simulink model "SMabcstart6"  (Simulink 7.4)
settings: Solver=ode45  StartTime=0.0  StopTime=10  MaxStep=2e-4  RelTol=1e-3
InitFcn:
  | smparamstart6
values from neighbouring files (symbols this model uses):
  Bm = 0.10    (= 0.1)    [IMabc2.m]    (also in imabcparam.m = 0.01; IMabcrun0.m = 0.01; IMabcrun1.m = 0.001; IMcur0.m = 1e-06)
  D = str2num(get(h,'string'))    [acttrcalc1.m]
  gam = 2*pi/3    (= 2.09439510239)    [IMabc2.m]    (also in IMabcf0.m; IMabcf1.m; imabcparam.m; IMabcrun0.m)
  H = 0.60    (= 0.6)    [IMabc2.m]    (also in IMcur0.m = 0.3; imdef0vec.m = 0.3; imdef1vec.m = 0.3; imdef2vec.m = 0.3)
  Lrr = [Lr   -Lm/2 -Lm/2    [IMabc2.m]    (also in IMabcf0.m = [Lr   -Lm1/2 -Lm1/2; IMabcf1.m = [Lr   -Lm1/2 -Lm1/2)
  Vm = Vll*sqrt(2/3)    [imabcparam.m]
  wo = 2*pi*freq0    [calc0.m]    (also in IMabc2.m = 376.991118431; imabcparam.m = 376.991118431; IMabcrun0.m = 376.991118431; IMabcrun1.m = 376.991118431)
undefined symbols (not defined in the file or in its folder): L2, Labo, Laf, Lakd, Lakq, Lao, R1, R2, Row, TL1, TL2, vector

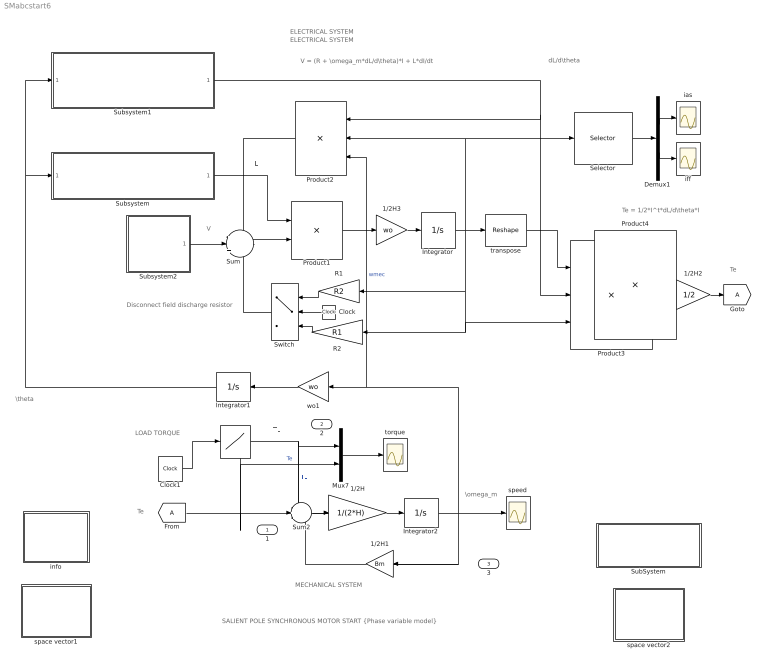
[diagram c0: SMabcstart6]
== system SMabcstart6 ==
  note: I
  note: I'
  note: MECHANICAL SYSTEM
  note: ELECTRICAL SYSTEM
  note: V
  note: SALIENT POLE SYNCHRONOUS MOTOR START {Phase variable model}
  note: L
  note: Te
  note: TL
  note: Te
  note: LOAD TORQUE
  note: Disconnect field discharge resistor
  note: dL/d\theta
  note: ELECTRICAL SYSTEM
  note: V = (R + \omega_m*dL/d\theta)*I + L*dI/dt
  note: \omega_m
  note: \theta
  note: Te = 1/2*I^t*dL/d\theta*I
  " " : Lookup  InputValues=[0 8 8 10 ]  Table="[TL1 TL1  TL2  TL2]"  OutDataType=sfix(16)  OutScaling=2^0
  1/2H : Gain  Gain=1/(2*H)  ParameterDataType=sfix(16)  ParameterScaling=2^0  OutDataType=sfix(16)  OutScaling=2^0
  1/2H1 : Gain  Gain=Bm  ParameterDataType=sfix(16)  ParameterScaling=2^0  OutDataType=sfix(16)  OutScaling=2^0
  1/2H2 : Gain  Gain=1/2  ParameterDataType=sfix(16)  ParameterScaling=2^0  OutDataType=sfix(16)  OutScaling=2^0
  1/2H3 : Gain  Gain=wo  ParameterDataType=sfix(16)  ParameterScaling=2^0  OutDataType=sfix(16)  OutScaling=2^0
  Clock : Clock
  Clock1 : Clock
  Demux1 : Demux  Outputs=2
  Integrator : Integrator  InitialCondition=[0 ;0 ;0; 0 ;0 ;0]
  Integrator1 : Integrator
  Integrator2 : Integrator
  Mux7 : Mux  Inputs=2
  Product1 : Product  Inputs=/*  Multiplication=Matrix(*)  OutDataType=sfix(16)  OutScaling=2^0
  Product2 : Product  Inputs=***  Multiplication=Matrix(*)  OutDataType=sfix(16)  OutScaling=2^0
  Product3 : Product  Inputs=3  Multiplication=Matrix(*)  OutDataType=sfix(16)  OutScaling=2^0
  Product4 : Product  Inputs=3  Multiplication=Matrix(*)  OutDataType=sfix(16)  OutScaling=2^0
  R1 : Gain  Gain=R2  Multiplication=Matrix(K*u)  ParameterDataType=sfix(16)  ParameterScaling=2^0  OutDataType=sfix(16)  OutScaling=2^0
  R2 : Gain  Gain=R1  Multiplication=Matrix(K*u)  ParameterDataType=sfix(16)  ParameterScaling=2^0  OutDataType=sfix(16)  OutScaling=2^0
  Selector : Selector  InputPortWidth=6  IndexOptions=Index vector (dialog)  Indices=[1 4]  OutputSizes=1
  SubSystem : Subsystem
  Subsystem : Subsystem
  Subsystem1 : Subsystem
  Subsystem2 : Subsystem
  Sum : Sum  Inputs=-|+|-  OutDataType=sfix(16)  OutScaling=2^0
  Sum2 : Sum  Inputs=-+-  OutDataType=sfix(16)  OutScaling=2^0
  Switch : Switch  Threshold=4
  ias : Scope
  iff : Scope
  info : Subsystem
  space vector1 : Subsystem
  space vector2 : Subsystem
  speed : Scope
  torque : Scope
  transpose : Reshape  OutputDimensionality=Row vector (2-D)  OutputDimensions=[1,6]
  wo1 : Gain  Gain=wo  ParameterDataType=sfix(16)  ParameterScaling=2^0  OutDataType=sfix(16)  OutScaling=2^0
  1 : Outport
  2 : Outport  Port=2
  3 : Outport  Port=3
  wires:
  Product1/1 -> 1/2H3/1
  Sum/1 -> Product1/2
  transpose/1 -> Product3/1
  Product2/1 -> Sum/1
  Subsystem1/1(dLdtheta) -> Product2/1, Product3/2
  Product3/1 -> 1/2H2/1
  Sum2/1 -> 1/2H/1
  1/2H/1 -> Integrator2/1
  1/2H1/1 -> Sum2/3
  Mux7/1 -> torque/1
  " "/1 -> Mux7/1, Sum2/1, 2/1  "TL"
  [A] -> Sum2/2, 1/1, Mux7/2  "Te"
  Integrator2/1 -> Product2/3, wo1/1, speed/1, 1/2H1/1, 3/1  "wmec"
  Subsystem2/1(V) -> Sum/2
  Integrator1/1 -> Subsystem1/1(theta1), Subsystem/1(theta)
  Clock1/1 -> " "/1
  1/2H2/1 -> [A]
  Subsystem/1(L) -> Product1/1
  R2/1 -> Switch/3
  R1/1 -> Switch/1
  Clock/1 -> Switch/2
  Switch/1 -> Sum/3
  Integrator/1 -> transpose/1, Product2/2, Selector/1, Product3/3, R2/1, R1/1
  Selector/1 -> Demux1/1
  Demux1/2 -> iff/1
  Demux1/1 -> ias/1
  1/2H3/1 -> Integrator/1
  wo1/1 -> Integrator1/1

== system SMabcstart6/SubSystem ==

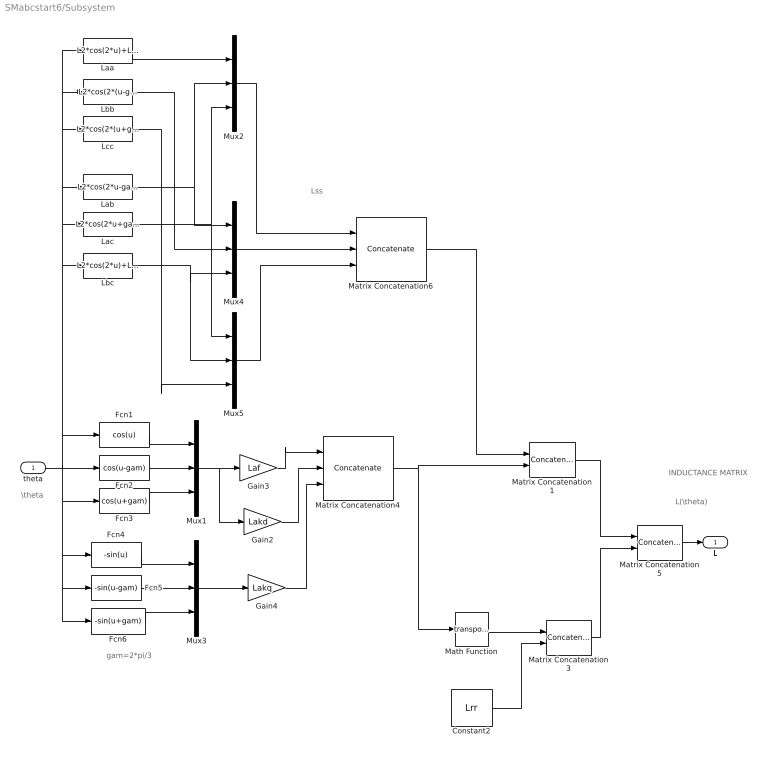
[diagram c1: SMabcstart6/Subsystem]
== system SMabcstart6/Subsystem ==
  note: INDUCTANCE MATRIX
  note: Lss
  note: L(\theta)
  note: gam=2*pi/3
  note: \theta
  theta : Inport  OutDataType=sfix(16)  OutScaling=2^0
  Constant2 : Constant  Value=Lrr  VectorParams1D=off  OutDataType=sfix(16)  OutScaling=2^0
  Fcn1 : Fcn  Expr=cos(u)
  Fcn2 : Fcn  Expr=cos(u-gam)
  Fcn3 : Fcn  Expr=cos(u+gam)
  Fcn4 : Fcn  Expr=-sin(u)
  Fcn5 : Fcn  Expr=-sin(u-gam)
  Fcn6 : Fcn  Expr=-sin(u+gam)
  Gain2 : Gain  Gain=Lakd  ParameterDataType=sfix(16)  ParameterScaling=2^0  OutDataType=sfix(16)  OutScaling=2^0
  Gain3 : Gain  Gain=Laf  ParameterDataType=sfix(16)  ParameterScaling=2^0  OutDataType=sfix(16)  OutScaling=2^0
  Gain4 : Gain  Gain=Lakq  ParameterDataType=sfix(16)  ParameterScaling=2^0  OutDataType=sfix(16)  OutScaling=2^0
  Laa : Fcn  Expr=L2*cos(2*u)+Lao
  Lab : Fcn  Expr=L2*cos(2*u-gam)+Labo
  Lac : Fcn  Expr=L2*cos(2*u+gam)+Labo
  Lbb : Fcn  Expr=L2*cos(2*(u-gam))+Lao
  Lbc : Fcn  Expr=L2*cos(2*u)+Labo
  Lcc : Fcn  Expr=L2*cos(2*(u+gam))+Lao
  Math Function : Math  Operator=transpose
  Matrix Concatenation1 : Concatenate  Mode=Multidimensional array  ConcatenateDimension=2
  Matrix Concatenation3 : Concatenate  Mode=Multidimensional array  ConcatenateDimension=2
  Matrix Concatenation4 : Concatenate  NumInputs=3  Mode=Multidimensional array  ConcatenateDimension=2
  Matrix Concatenation5 : Concatenate  Mode=Multidimensional array
  Matrix Concatenation6 : Concatenate  NumInputs=3  Mode=Multidimensional array  ConcatenateDimension=2
  Mux{1..5} (5 alike) : Mux  Inputs=3
  L : Outport
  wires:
  Matrix Concatenation5/1 -> L/1
  Matrix Concatenation4/1 -> Matrix Concatenation1/2, Math Function/1
  Mux1/1 -> Gain3/1, Gain2/1
  Matrix Concatenation1/1 -> Matrix Concatenation5/1
  Fcn3/1 -> Mux1/3
  Fcn2/1 -> Mux1/2
  Fcn1/1 -> Mux1/1
  theta/1 -> Fcn2/1, Fcn3/1, Fcn6/1, Fcn5/1, Fcn4/1, Fcn1/1, Laa/1, Lbb/1, Lcc/1, Lab/1, Lac/1, Lbc/1
  Gain3/1 -> Matrix Concatenation4/1
  Gain2/1 -> Matrix Concatenation4/2
  Fcn5/1 -> Mux3/2
  Fcn4/1 -> Mux3/1
  Fcn6/1 -> Mux3/3
  Mux3/1 -> Gain4/1
  Gain4/1 -> Matrix Concatenation4/3
  Constant2/1 -> Matrix Concatenation3/2
  Matrix Concatenation3/1 -> Matrix Concatenation5/2
  Laa/1 -> Mux2/1
  Lbb/1 -> Mux4/2
  Lab/1 -> Mux2/2, Mux4/1
  Lac/1 -> Mux2/3, Mux5/1
  Lbc/1 -> Mux4/3, Mux5/2
  Lcc/1 -> Mux5/3
  Mux4/1 -> Matrix Concatenation6/2
  Mux2/1 -> Matrix Concatenation6/1
  Mux5/1 -> Matrix Concatenation6/3
  Matrix Concatenation6/1 -> Matrix Concatenation1/1
  Math Function/1 -> Matrix Concatenation3/1

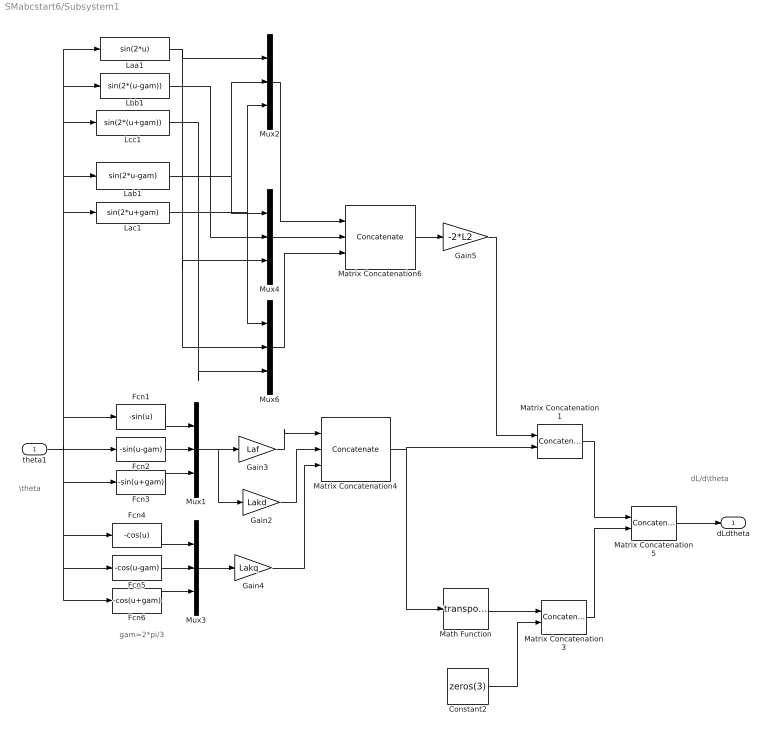
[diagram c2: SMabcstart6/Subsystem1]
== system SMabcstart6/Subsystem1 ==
  note: dL/d\theta
  note: \theta
  note: gam=2*pi/3
  theta1 : Inport  OutDataType=sfix(16)  OutScaling=2^0
  Constant2 : Constant  Value=zeros(3)  VectorParams1D=off  OutDataType=sfix(16)  OutScaling=2^0
  Fcn1 : Fcn  Expr=-sin(u)
  Fcn2 : Fcn  Expr=-sin(u-gam)
  Fcn3 : Fcn  Expr=-sin(u+gam)
  Fcn4 : Fcn  Expr=-cos(u)
  Fcn5 : Fcn  Expr=-cos(u-gam)
  Fcn6 : Fcn  Expr=-cos(u+gam)
  Gain2 : Gain  Gain=Lakd  ParameterDataType=sfix(16)  ParameterScaling=2^0  OutDataType=sfix(16)  OutScaling=2^0
  Gain3 : Gain  Gain=Laf  ParameterDataType=sfix(16)  ParameterScaling=2^0  OutDataType=sfix(16)  OutScaling=2^0
  Gain4 : Gain  Gain=Lakq  ParameterDataType=sfix(16)  ParameterScaling=2^0  OutDataType=sfix(16)  OutScaling=2^0
  Gain5 : Gain  Gain=-2*L2  ParameterDataType=sfix(16)  ParameterScaling=2^0  OutDataType=sfix(16)  OutScaling=2^0
  Laa1 : Fcn  Expr=sin(2*u)
  Lab1 : Fcn  Expr=sin(2*u-gam)
  Lac1 : Fcn  Expr=sin(2*u+gam)
  Lbb1 : Fcn  Expr=sin(2*(u-gam))
  Lcc1 : Fcn  Expr=sin(2*(u+gam))
  Math Function : Math  Operator=transpose
  Matrix Concatenation1 : Concatenate  Mode=Multidimensional array  ConcatenateDimension=2
  Matrix Concatenation3 : Concatenate  Mode=Multidimensional array  ConcatenateDimension=2
  Matrix Concatenation4 : Concatenate  NumInputs=3  Mode=Multidimensional array  ConcatenateDimension=2
  Matrix Concatenation5 : Concatenate  Mode=Multidimensional array
  Matrix Concatenation6 : Concatenate  NumInputs=3  Mode=Multidimensional array  ConcatenateDimension=2
  Mux{1..4,6} (5 alike) : Mux  Inputs=3
  dLdtheta : Outport
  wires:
  Matrix Concatenation5/1 -> dLdtheta/1
  Matrix Concatenation4/1 -> Matrix Concatenation1/2, Math Function/1
  Mux1/1 -> Gain3/1, Gain2/1
  Matrix Concatenation1/1 -> Matrix Concatenation5/1
  Fcn3/1 -> Mux1/3
  Fcn2/1 -> Mux1/2
  Fcn1/1 -> Mux1/1
  theta1/1 -> Fcn2/1, Fcn3/1, Fcn6/1, Fcn5/1, Fcn4/1, Fcn1/1, Laa1/1, Lbb1/1, Lcc1/1, Lab1/1, Lac1/1
  Gain3/1 -> Matrix Concatenation4/1
  Gain2/1 -> Matrix Concatenation4/2
  Fcn5/1 -> Mux3/2
  Fcn4/1 -> Mux3/1
  Fcn6/1 -> Mux3/3
  Mux3/1 -> Gain4/1
  Gain4/1 -> Matrix Concatenation4/3
  Constant2/1 -> Matrix Concatenation3/2
  Matrix Concatenation3/1 -> Matrix Concatenation5/2
  Laa1/1 -> Mux2/1, Mux4/3, Mux6/2
  Lbb1/1 -> Mux4/2
  Lab1/1 -> Mux2/2, Mux4/1
  Lac1/1 -> Mux2/3, Mux6/1
  Lcc1/1 -> Mux6/3
  Mux4/1 -> Matrix Concatenation6/2
  Mux2/1 -> Matrix Concatenation6/1
  Mux6/1 -> Matrix Concatenation6/3
  Matrix Concatenation6/1 -> Gain5/1
  Gain5/1 -> Matrix Concatenation1/1
  Math Function/1 -> Matrix Concatenation3/1

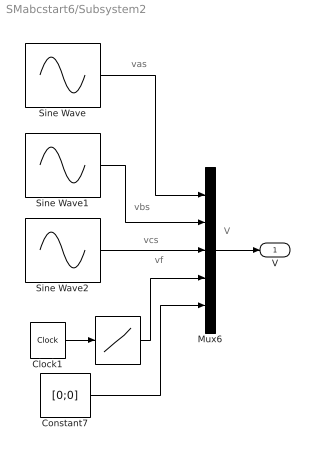
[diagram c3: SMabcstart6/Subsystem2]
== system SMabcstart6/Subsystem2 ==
  note: V
  note: vf
  note: vcs
  note: vbs
  note: vas
  " " : Lookup  InputValues=[0 4 4 10 ]  Table="[0  0  .02  0.02]"  OutDataType=sfix(16)  OutScaling=2^0
  Clock1 : Clock
  Constant7 : Constant  Value=[0;0]  VectorParams1D=off  OutDataType=sfix(16)  OutScaling=2^0
  Mux6 : Mux  Inputs=5
  Sine Wave : Sin  Amplitude=Vm  Bias=0  Frequency=wo  Phase=pi/2  Samples=10  SampleTime=0
  Sine Wave1 : Sin  Amplitude=Vm  Bias=0  Frequency=wo  Phase=pi/2-gam  Samples=10  SampleTime=0
  Sine Wave2 : Sin  Amplitude=Vm  Bias=0  Frequency=wo  Phase=pi/2+gam  Samples=10  SampleTime=0
  V : Outport
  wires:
  Mux6/1 -> V/1
  Sine Wave2/1 -> Mux6/3
  Sine Wave1/1 -> Mux6/2
  Sine Wave/1 -> Mux6/1
  Constant7/1 -> Mux6/5
  Clock1/1 -> " "/1
  " "/1 -> Mux6/4

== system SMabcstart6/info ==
  note: START OF A SALIENT POLE SYNCHRONOUS MOTOR (Phase variable model) [pu]
  note: A salient pole synchronous motor is started from stanstill at rated voltage with the dc field circuit shorted across an external field discharge resistor. When synchronous is almost attained, the discharge resistor is removed and a dc voltage is applied to the field circuit so that the motor will now run at synchronous speed. A load torque is then suddenly applied. The dynamic equations are expressed in matrix form in terms the phase variables, namely the stator currents ias, ibs, ics; the rotor field current iff; the d-axis and q-axis damper currents idk and iqk; the anglar speed wm; and the displacement angle theta between stator as-axis and rotor direct axis. Torque, speed and current responses are plotted. A Matlab script file for the identical system operation is given in the file >.

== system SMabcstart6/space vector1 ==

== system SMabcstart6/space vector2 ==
